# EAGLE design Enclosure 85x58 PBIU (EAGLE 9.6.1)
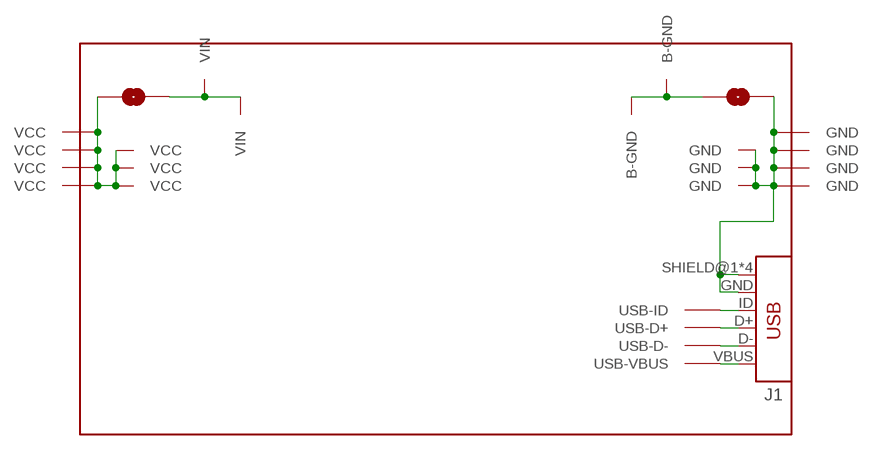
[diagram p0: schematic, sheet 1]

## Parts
J1  USB_MINI-B_SMT  [USB-MINIB]
U$1  PROTO-28X18-BAT-USB-SJ  [PROTO-28X18-BAT-USB-SJ]

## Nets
GND: J1.GND J1.SHIELD@1(SHIELD) J1.SHIELD@2(SHIELD) J1.SHIELD@3(SHIELD) J1.SHIELD@4(SHIELD) U$1.GND U$1.P27-11(GND) U$1.P27-12(GND) U$1.P27-13(GND) U$1.P28-11(GND) U$1.P28-12(GND) U$1.P28-13(GND) U$1.P28-14(GND)
N$2: U$1.P02-14(VIN) U$1.P03-14(VIN) U$1.VIN
N$3: U$1.B-GND U$1.P25-14(B-GND) U$1.P27-14(B-GND)
N$5: J1.VBUS U$1.P25-04(USB-VBUS)
N$6: J1.D- U$1.P25-05(USB-D-)
N$7: J1.D+ U$1.P25-06(USB-D+)
N$8: J1.ID U$1.P25-07(USB-ID)
VCC: U$1.P01-11(VCC) U$1.P01-12(VCC) U$1.P01-13(VCC) U$1.P01-14(VCC) U$1.P02-11(VCC) U$1.P02-12(VCC) U$1.P02-13(VCC) U$1.VCC

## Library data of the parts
J1 = digitalconcepts:USB_MINI-B: USB Mini-B Connector Breaks out 5 pins, and includes shield pins if needed.
U$1 = digitalconcepts:PROTO-28X18-BAT-USB-SJ: 28 x 18 Prototyping board, with SJ between battery connections and GND/Vcc planes and coupled side connection points, to fit an 85 x 58 enclosure

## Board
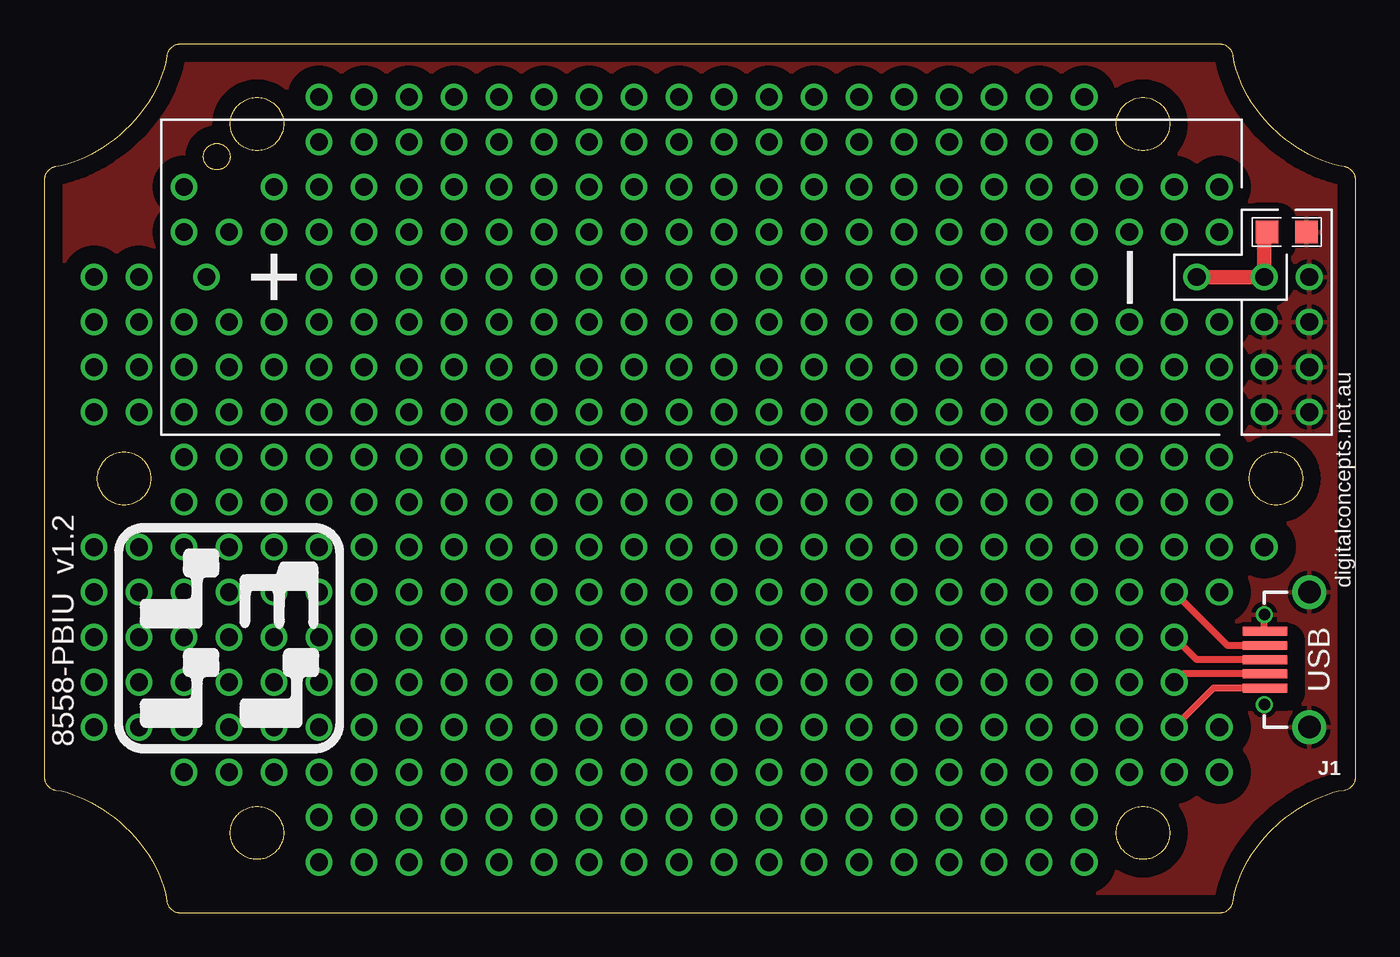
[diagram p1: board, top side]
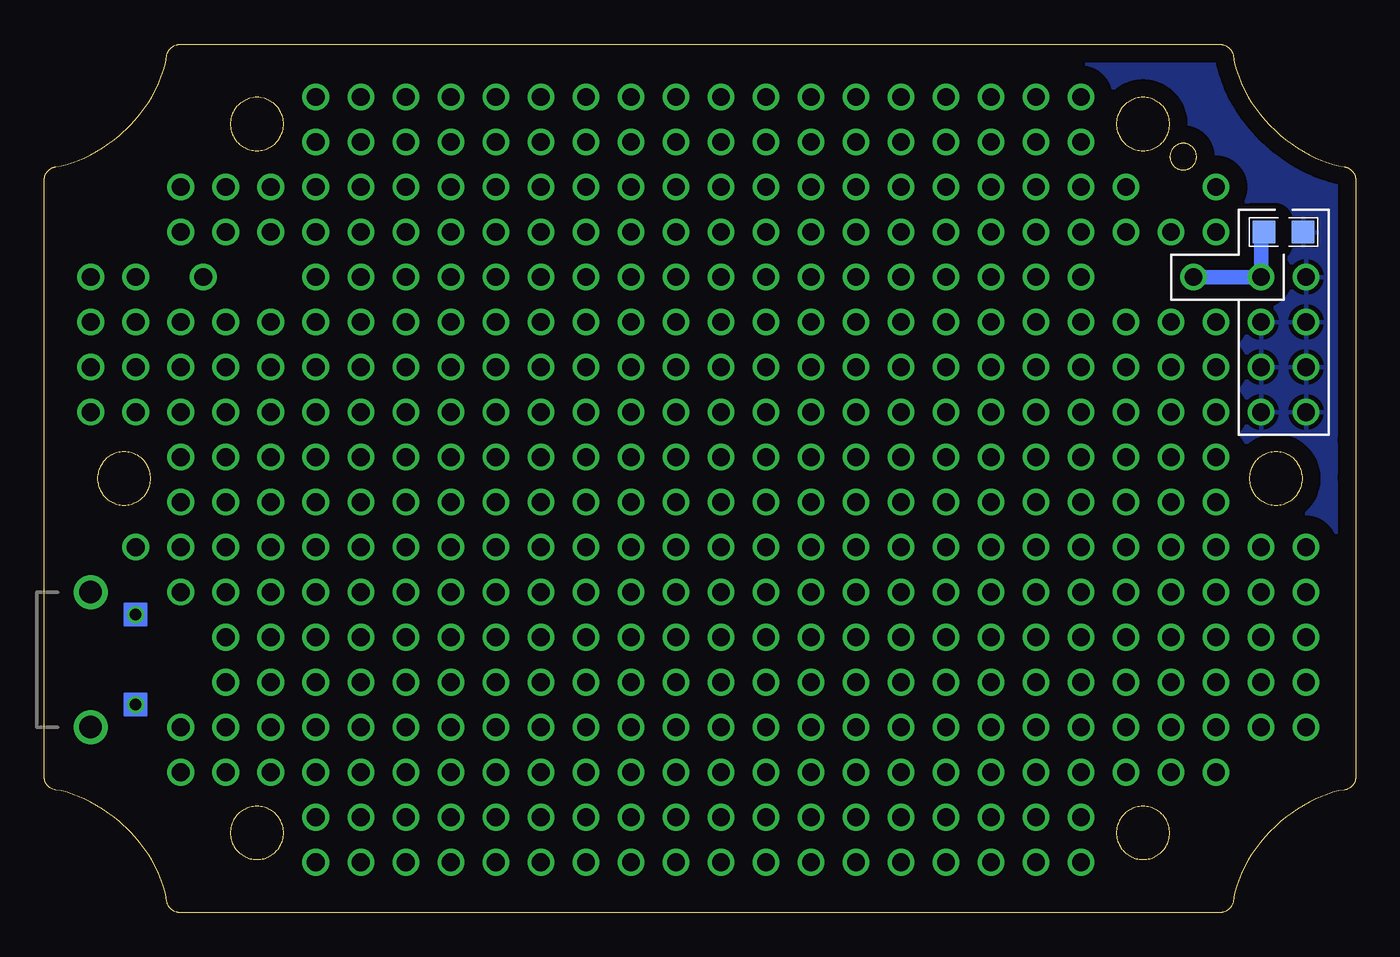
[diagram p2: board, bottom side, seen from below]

Size 74 x 49 mm. Coordinates in mm from the lower left corner, seen from the top.
Outline: 909 segments
Copper layers (1*16): Top 0.035mm / dielectric 1.5mm / Bottom 0.035mm
Design rules "default *": minimum track width 6mil, minimum drill 0.35mm, track to track 6mil, track to pad 6mil, pad to pad 6mil, via to via 6mil, smd to smd 6mil, copper to edge 40mil, drill to drill 6mil, minimum pad ring 1mil, minimum via ring 8mil, stop-mask expansion 4mil, vias tented up to drill 0mil, thermal gap 10mil

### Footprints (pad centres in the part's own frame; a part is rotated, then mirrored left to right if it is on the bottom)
USB-MINIB = smd 2.5 x 0.5: D+ 2.5,0; D- 2.5,0.8; GND 2.5,-1.6; ID 2.5,-0.8; VBUS 2.5,1.6 | drill 1.27: SHIELD@1 0,3.81; SHIELD@2 0,-3.81 | drill 0.65 pad 0.762: SHIELD@3 2.54,2.54; SHIELD@4 2.54,-2.54
PROTO-28X18-BAT-USB-SJ = smd 1.27 x 1.27: B-GND 31.914,13.97; GND 34.126,13.97 | drill 1: P01-04 -34.29,-13.97; P01-05 -34.29,-11.43; P01-06 -34.29,-8.89; P01-07 -34.29,-6.35; P01-08 -34.29,-3.81; P01-11 -34.29,3.81; P01-12 -34.29,6.35; P01-13 -34.29,8.89; P01-14 -34.29,11.43; P02-04 -31.75,-13.97; P02-05 -31.75,-11.43; P02-06 -31.75,-8.89; P02-07 -31.75,-6.35; P02-08 -31.75,-3.81; P02-11 -31.75,3.81; P02-12 -31.75,6.35; P02-13 -31.75,8.89; P02-14 -31.75,11.43; P03-03 -29.21,-16.51; P03-04 -29.21,-13.97; P03-05 -29.21,-11.43; P03-06 -29.21,-8.89; P03-07 -29.21,-6.35; P03-08 -29.21,-3.81; P03-09 -29.21,-1.27; P03-10 -29.21,1.27; P03-11 -29.21,3.81; P03-12 -29.21,6.35; P03-13 -29.21,8.89; P03-14 -27.94,11.43; P03-15 -29.21,13.97; P03-16 -29.21,16.51; P04-03 -26.67,-16.51; P04-04 -26.67,-13.97; P04-05 -26.67,-11.43; P04-06 -26.67,-8.89; P04-07 -26.67,-6.35; P04-08 -26.67,-3.81; P04-09 -26.67,-1.27; P04-10 -26.67,1.27; P04-11 -26.67,3.81; P04-12 -26.67,6.35; P04-13 -26.67,8.89; P04-15 -26.67,13.97; P05-03 -24.13,-16.51; P05-04 -24.13,-13.97; P05-05 -24.13,-11.43; P05-06 -24.13,-8.89; P05-07 -24.13,-6.35; P05-08 -24.13,-3.81; P05-09 -24.13,-1.27; P05-10 -24.13,1.27; P05-11 -24.13,3.81; P05-12 -24.13,6.35; P05-13 -24.13,8.89; P05-15 -24.13,13.97; P05-16 -24.13,16.51; P06-01 -21.59,-21.59; P06-02 -21.59,-19.05; P06-03 -21.59,-16.51; P06-04 -21.59,-13.97; P06-05 -21.59,-11.43; P06-06 -21.59,-8.89; P06-07 -21.59,-6.35; P06-08 -21.59,-3.81; P06-09 -21.59,-1.27; P06-10 -21.59,1.27; P06-11 -21.59,3.81; P06-12 -21.59,6.35; P06-13 -21.59,8.89; P06-14 -21.59,11.43; P06-15 -21.59,13.97; P06-16 -21.59,16.51; P06-17 -21.59,19.05; P06-18 -21.59,21.59; P07-01 -19.05,-21.59; P07-02 -19.05,-19.05; P07-03 -19.05,-16.51; P07-04 -19.05,-13.97; P07-05 -19.05,-11.43; P07-06 -19.05,-8.89; P07-07 -19.05,-6.35; P07-08 -19.05,-3.81; P07-09 -19.05,-1.27; P07-10 -19.05,1.27; P07-11 -19.05,3.81; P07-12 -19.05,6.35; P07-13 -19.05,8.89; P07-14 -19.05,11.43; P07-15 -19.05,13.97; P07-16 -19.05,16.51; P07-17 -19.05,19.05; P07-18 -19.05,21.59; P08-01 -16.51,-21.59; P08-02 -16.51,-19.05; P08-03 -16.51,-16.51; P08-04 -16.51,-13.97; P08-05 -16.51,-11.43; P08-06 -16.51,-8.89; P08-07 -16.51,-6.35; P08-08 -16.51,-3.81; P08-09 -16.51,-1.27; P08-10 -16.51,1.27; P08-11 -16.51,3.81; P08-12 -16.51,6.35; P08-13 -16.51,8.89; P08-14 -16.51,11.43; P08-15 -16.51,13.97; P08-16 -16.51,16.51; P08-17 -16.51,19.05; P08-18 -16.51,21.59; P09-01 -13.97,-21.59; P09-02 -13.97,-19.05; P09-03 -13.97,-16.51; P09-04 -13.97,-13.97; P09-05 -13.97,-11.43; P09-06 -13.97,-8.89; P09-07 -13.97,-6.35; P09-08 -13.97,-3.81; P09-09 -13.97,-1.27; P09-10 -13.97,1.27; P09-11 -13.97,3.81; P09-12 -13.97,6.35; P09-13 -13.97,8.89; P09-14 -13.97,11.43; P09-15 -13.97,13.97; P09-16 -13.97,16.51; P09-17 -13.97,19.05; P09-18 -13.97,21.59; P10-01 -11.43,-21.59; P10-02 -11.43,-19.05; P10-03 -11.43,-16.51; P10-04 -11.43,-13.97; P10-05 -11.43,-11.43; P10-06 -11.43,-8.89; P10-07 -11.43,-6.35; P10-08 -11.43,-3.81; P10-09 -11.43,-1.27; P10-10 -11.43,1.27; P10-11 -11.43,3.81; P10-12 -11.43,6.35; P10-13 -11.43,8.89; P10-14 -11.43,11.43; P10-15 -11.43,13.97; P10-16 -11.43,16.51; P10-17 -11.43,19.05; P10-18 -11.43,21.59; P11-01 -8.89,-21.59; P11-02 -8.89,-19.05; P11-03 -8.89,-16.51; P11-04 -8.89,-13.97; P11-05 -8.89,-11.43; P11-06 -8.89,-8.89; P11-07 -8.89,-6.35; P11-08 -8.89,-3.81; P11-09 -8.89,-1.27; P11-10 -8.89,1.27; P11-11 -8.89,3.81; P11-12 -8.89,6.35; P11-13 -8.89,8.89; P11-14 -8.89,11.43; P11-15 -8.89,13.97; P11-16 -8.89,16.51; P11-17 -8.89,19.05; P11-18 -8.89,21.59; P12-01 -6.35,-21.59; P12-02 -6.35,-19.05; P12-03 -6.35,-16.51; P12-04 -6.35,-13.97; P12-05 -6.35,-11.43; P12-06 -6.35,-8.89; P12-07 -6.35,-6.35; P12-08 -6.35,-3.81; P12-09 -6.35,-1.27; P12-10 -6.35,1.27; P12-11 -6.35,3.81; P12-12 -6.35,6.35; P12-13 -6.35,8.89; P12-14 -6.35,11.43; P12-15 -6.35,13.97; P12-16 -6.35,16.51; P12-17 -6.35,19.05; P12-18 -6.35,21.59; P13-01 -3.81,-21.59; P13-02 -3.81,-19.05; P13-03 -3.81,-16.51; P13-04 -3.81,-13.97; P13-05 -3.81,-11.43; P13-06 -3.81,-8.89; P13-07 -3.81,-6.35; P13-08 -3.81,-3.81; P13-09 -3.81,-1.27; P13-10 -3.81,1.27; P13-11 -3.81,3.81; P13-12 -3.81,6.35; P13-13 -3.81,8.89; P13-14 -3.81,11.43; P13-15 -3.81,13.97; P13-16 -3.81,16.51; P13-17 -3.81,19.05; P13-18 -3.81,21.59; P14-01 -1.27,-21.59; P14-02 -1.27,-19.05; P14-03 -1.27,-16.51; P14-04 -1.27,-13.97; P14-05 -1.27,-11.43; P14-06 -1.27,-8.89; P14-07 -1.27,-6.35; P14-08 -1.27,-3.81; P14-09 -1.27,-1.27; P14-10 -1.27,1.27; P14-11 -1.27,3.81; P14-12 -1.27,6.35; P14-13 -1.27,8.89; P14-14 -1.27,11.43; P14-15 -1.27,13.97; P14-16 -1.27,16.51; P14-17 -1.27,19.05; P14-18 -1.27,21.59; P15-01 1.27,-21.59; P15-02 1.27,-19.05; P15-03 1.27,-16.51; P15-04 1.27,-13.97; P15-05 1.27,-11.43; P15-06 1.27,-8.89; P15-07 1.27,-6.35; P15-08 1.27,-3.81; P15-09 1.27,-1.27; P15-10 1.27,1.27; P15-11 1.27,3.81; P15-12 1.27,6.35; P15-13 1.27,8.89; P15-14 1.27,11.43; P15-15 1.27,13.97; P15-16 1.27,16.51; P15-17 1.27,19.05; P15-18 1.27,21.59; P16-01 3.81,-21.59; P16-02 3.81,-19.05; P16-03 3.81,-16.51; P16-04 3.81,-13.97; P16-05 3.81,-11.43; P16-06 3.81,-8.89; P16-07 3.81,-6.35; P16-08 3.81,-3.81; P16-09 3.81,-1.27; P16-10 3.81,1.27; P16-11 3.81,3.81; P16-12 3.81,6.35; P16-13 3.81,8.89; P16-14 3.81,11.43; P16-15 3.81,13.97; P16-16 3.81,16.51; P16-17 3.81,19.05; P16-18 3.81,21.59; P17-01 6.35,-21.59; P17-02 6.35,-19.05; P17-03 6.35,-16.51; P17-04 6.35,-13.97; P17-05 6.35,-11.43; P17-06 6.35,-8.89; P17-07 6.35,-6.35; P17-08 6.35,-3.81; P17-09 6.35,-1.27; P17-10 6.35,1.27; P17-11 6.35,3.81; P17-12 6.35,6.35; P17-13 6.35,8.89; P17-14 6.35,11.43; P17-15 6.35,13.97; P17-16 6.35,16.51; P17-17 6.35,19.05; P17-18 6.35,21.59; P18-01 8.89,-21.59; P18-02 8.89,-19.05; P18-03 8.89,-16.51; P18-04 8.89,-13.97; P18-05 8.89,-11.43; P18-06 8.89,-8.89; P18-07 8.89,-6.35; P18-08 8.89,-3.81; P18-09 8.89,-1.27; P18-10 8.89,1.27; P18-11 8.89,3.81; P18-12 8.89,6.35; P18-13 8.89,8.89; P18-14 8.89,11.43; P18-15 8.89,13.97; P18-16 8.89,16.51; P18-17 8.89,19.05; P18-18 8.89,21.59; P19-01 11.43,-21.59; P19-02 11.43,-19.05; P19-03 11.43,-16.51; P19-04 11.43,-13.97; P19-05 11.43,-11.43; P19-06 11.43,-8.89; P19-07 11.43,-6.35; P19-08 11.43,-3.81; P19-09 11.43,-1.27; P19-10 11.43,1.27; P19-11 11.43,3.81; P19-12 11.43,6.35; P19-13 11.43,8.89; P19-14 11.43,11.43; P19-15 11.43,13.97; P19-16 11.43,16.51; P19-17 11.43,19.05; P19-18 11.43,21.59; P20-01 13.97,-21.59; P20-02 13.97,-19.05; P20-03 13.97,-16.51; P20-04 13.97,-13.97; P20-05 13.97,-11.43; P20-06 13.97,-8.89; P20-07 13.97,-6.35; P20-08 13.97,-3.81; P20-09 13.97,-1.27; P20-10 13.97,1.27; P20-11 13.97,3.81; P20-12 13.97,6.35; P20-13 13.97,8.89; P20-14 13.97,11.43; P20-15 13.97,13.97; P20-16 13.97,16.51; P20-17 13.97,19.05; P20-18 13.97,21.59; P21-01 16.51,-21.59; P21-02 16.51,-19.05; P21-03 16.51,-16.51; P21-04 16.51,-13.97; P21-05 16.51,-11.43; P21-06 16.51,-8.89; P21-07 16.51,-6.35; P21-08 16.51,-3.81; P21-09 16.51,-1.27; P21-10 16.51,1.27; P21-11 16.51,3.81; P21-12 16.51,6.35; P21-13 16.51,8.89; P21-14 16.51,11.43; P21-15 16.51,13.97; P21-16 16.51,16.51; P21-17 16.51,19.05; P21-18 16.51,21.59; P22-01 19.05,-21.59; P22-02 19.05,-19.05; P22-03 19.05,-16.51; P22-04 19.05,-13.97; P22-05 19.05,-11.43; P22-06 19.05,-8.89; P22-07 19.05,-6.35; P22-08 19.05,-3.81; P22-09 19.05,-1.27; P22-10 19.05,1.27; P22-11 19.05,3.81; P22-12 19.05,6.35; P22-13 19.05,8.89; P22-14 19.05,11.43; P22-15 19.05,13.97; P22-16 19.05,16.51; P22-17 19.05,19.05; P22-18 19.05,21.59; P23-01 21.59,-21.59; P23-02 21.59,-19.05; P23-03 21.59,-16.51; P23-04 21.59,-13.97; P23-05 21.59,-11.43; P23-06 21.59,-8.89; P23-07 21.59,-6.35; P23-08 21.59,-3.81; P23-09 21.59,-1.27; P23-10 21.59,1.27; P23-11 21.59,3.81; P23-12 21.59,6.35; P23-13 21.59,8.89; P23-14 21.59,11.43; P23-15 21.59,13.97; P23-16 21.59,16.51; P23-17 21.59,19.05; P23-18 21.59,21.59; P24-03 24.13,-16.51; P24-04 24.13,-13.97; P24-05 24.13,-11.43; P24-06 24.13,-8.89; P24-07 24.13,-6.35; P24-08 24.13,-3.81; P24-09 24.13,-1.27; P24-10 24.13,1.27; P24-11 24.13,3.81; P24-12 24.13,6.35; P24-13 24.13,8.89; P24-15 24.13,13.97; P24-16 24.13,16.51; P25-03 26.67,-16.51; P25-04 26.67,-13.97; P25-05 26.67,-11.43; P25-06 26.67,-8.89; P25-07 26.67,-6.35; P25-08 26.67,-3.81; P25-09 26.67,-1.27; P25-10 26.67,1.27; P25-11 26.67,3.81; P25-12 26.67,6.35; P25-13 26.67,8.89; P25-14 27.94,11.43; P25-15 26.67,13.97; P25-16 26.67,16.51; P26-03 29.21,-16.51; P26-04 29.21,-13.97; P26-07 29.21,-6.35; P26-08 29.21,-3.81; P26-09 29.21,-1.27; P26-10 29.21,1.27; P26-11 29.21,3.81; P26-12 29.21,6.35; P26-13 29.21,8.89; P26-15 29.21,13.97; P26-16 29.21,16.51; P27-08 31.75,-3.81; P27-11 31.75,3.81; P27-12 31.75,6.35; P27-13 31.75,8.89; P27-14 31.75,11.43; P28-11 34.29,3.81; P28-12 34.29,6.35; P28-13 34.29,8.89; P28-14 34.29,11.43 | smd 1.27 x 1.27 bottom: VCC -34.126,13.97; VIN -31.914,13.97

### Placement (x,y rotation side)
J1  71.38,14.27 180 top
U$1  37.09,24.43 0 top

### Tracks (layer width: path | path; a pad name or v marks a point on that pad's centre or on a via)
GND
  Top 0.152: J1.GND 68.84,15.91
  Top 0.406: 68.84,15.91 J1.SHIELD@4
  pour Top (isolate 1.016): -1.26,50.34 75.19,50.34 75.19,-1.48 -1.26,-1.48
N$2
  Bottom 0.813: U$1.P03-14 U$1.P02-14 5.34,38.24 U$1.VIN
N$3
  Top 0.152: 68.84,38.24 U$1.B-GND
  Top 0.813: U$1.P25-14 U$1.P27-14 68.84,38.24
N$5
  Top 0.406: J1.VBUS 65.97,12.67 U$1.P25-04
N$6
  Top 0.406: J1.D- 64.23,13.47 U$1.P25-05
N$7
  Top 0.406: J1.D+ 65.03,14.27 U$1.P25-06
N$8
  Top 0.406: J1.ID 66.77,15.07 U$1.P25-07
VCC
  pour Bottom (isolate 1.016): 0.01,49.07 73.92,49.07 73.92,-0.21 0.01,-0.21

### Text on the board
tPlace: + | – | digitalconcepts.net.au | 8558-PBIU v1.2 | USB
